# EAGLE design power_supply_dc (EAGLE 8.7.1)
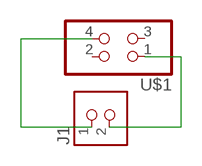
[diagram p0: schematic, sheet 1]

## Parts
J1  TERM-1X02-ADAFRUIT  [3.5MMTERM]
U$1  PINHD-2X2-SMD  [2X02SMD]

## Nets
N$1: J1.1 U$1.4
N$2: J1.2 U$1.1
Unconnected: U$1.2 U$1.3

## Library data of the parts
J1 = fab:TERM-1X02: 3.5mm terminal block, 2 positions ED555-2DS as found in the fablab inventory.
U$1 = fab:PINHD-2X2-SMD

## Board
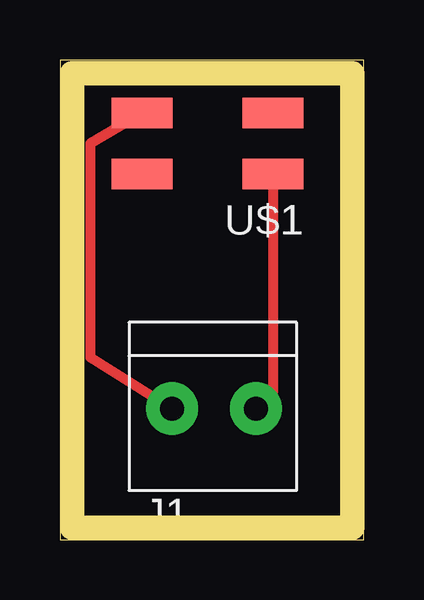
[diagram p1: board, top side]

Size 12.68 x 19.99 mm. Coordinates in mm from the lower left corner, seen from the top.
Outline: 0,0 12.68,0 12.68,19.99 0,19.99 0,0
Copper layers (1*16): Top 0.035mm / dielectric 1.5mm / Bottom 0.035mm
Design rules "default *": minimum track width 16mil, minimum drill 0.35mm, track to track 16mil, track to pad 16mil, pad to pad 16mil, via to via 16mil, smd to smd 16mil, copper to edge 40mil, drill to drill 16mil, minimum pad ring 10mil, minimum via ring 8mil, stop-mask expansion 4mil, vias tented up to drill 0mil, thermal gap 10mil
Milling: 4 lines

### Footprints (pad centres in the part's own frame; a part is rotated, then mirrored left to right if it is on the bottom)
3.5MMTERM = drill 1 pad 2.184: 1 1.8,0; 2 -1.7,0
2X02SMD = smd 2.54 x 1.27: 1 -2.54,1.27; 2 2.92,1.27; 3 -2.54,-1.27; 4 2.92,-1.27

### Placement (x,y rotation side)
J1  6.48,5.46 180 top
U$1  6.35,16.51 180 top

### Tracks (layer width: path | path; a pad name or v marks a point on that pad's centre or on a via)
N$1
  Top 0.406: U$1.4 1.27,16.51 1.27,7.6 J1.1
N$2
  Top 0.406: U$1.1 8.89,6.17 J1.2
